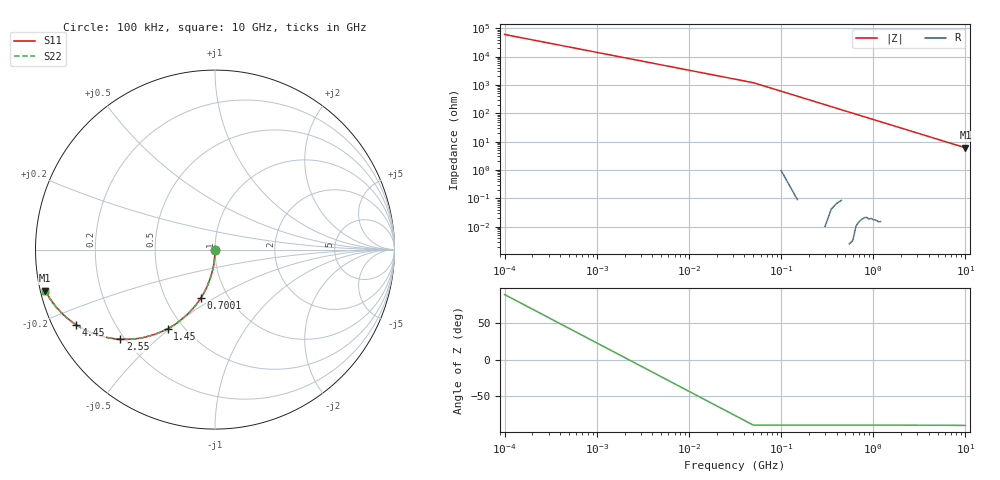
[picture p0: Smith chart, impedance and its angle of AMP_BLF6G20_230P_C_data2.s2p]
! Created Tue Aug  7 13:48:20 2007
# hz S ri R 50
! 2 Port Network Data from SP1.SP block
! freq  reS11  imS11  reS21  imS21  reS12  imS12  reS22  imS22
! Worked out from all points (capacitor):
!   201 points, 100 kHz to 10 GHz, reference 50 ohm
!   read as one part in shunt: C = 2.64 pF near 50.1 MHz
!   lowest |Z| = 6.09 ohm at 10 GHz (marker M1)
!   S11 on the Smith chart (normalised r, x): 100 kHz: 1.00, +0.00; 700.1 MHz: 0.75, -0.43; 1.45 GHz: 0.41, -0.49; 2.55 GHz: 0.18, -0.39; 4.45 GHz: 0.07, -0.25; 10 GHz: 0.01, -0.12
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100000  -2.85e-06 0.000389  1 0.000414  1 0.000414  -2.7e-06 0.000441
5.01e7  -0.000416 -0.0208  0.9996 -0.0209  0.9996 -0.0209  -0.000413 -0.0209
1.001e8  -0.00177 -0.0413  0.9982 -0.0415  0.9982 -0.0415  -0.00178 -0.0415
1.501e8  -0.00386 -0.0618  0.9961 -0.0621  0.9961 -0.0621  -0.00386 -0.0621
2.001e8  -0.00679 -0.082  0.9932 -0.0824  0.9932 -0.0824  -0.00679 -0.0824
2.501e8  -0.0106 -0.1021  0.9894 -0.1026  0.9894 -0.1026  -0.0106 -0.1025
3.001e8  -0.0152 -0.1219  0.9848 -0.1225  0.9848 -0.1225  -0.0152 -0.1224
4.001e8  -0.0267 -0.1606  0.9732 -0.1614  0.9732 -0.1614  -0.0267 -0.1612
5.001e8  -0.0411 -0.1991  0.9588 -0.1986  0.9588 -0.1986  -0.0411 -0.1984
7.001e8  -0.0775 -0.2676  0.9223 -0.2675  0.9223 -0.2675  -0.0775 -0.2672
8.501e8  -0.1103 -0.313  0.8896 -0.3133  0.8896 -0.3133  -0.1103 -0.313
1.0501e9  -0.1588 -0.365  0.841 -0.3657  0.841 -0.3657  -0.1588 -0.3653
1.4501e9  -0.2645 -0.4413  0.7352 -0.4415  0.7352 -0.4415  -0.2644 -0.441
1.7001e9  -0.3309 -0.4702  0.6688 -0.471  0.6688 -0.471  -0.3308 -0.4705
2.0501e9  -0.4183 -0.4937  0.5814 -0.4938  0.5814 -0.4938  -0.4181 -0.4933
2.5501e9  -0.5266 -0.5002  0.473 -0.5  0.473 -0.5  -0.5264 -0.4994
3.3501e9  -0.6575 -0.4752  0.3421 -0.4755  0.3421 -0.4755  -0.6572 -0.4749
4.4501e9  -0.7722 -0.4191  0.2274 -0.4207  0.2274 -0.4207  -0.7719 -0.4201
5.0001e9  -0.8106 -0.3919  0.1889 -0.3932  0.1889 -0.3932  -0.8102 -0.3926
6.7001e9  -0.885 -0.3203  0.1145 -0.3209  0.1145 -0.3209  -0.8846 -0.3203
8.3501e9  -0.923 -0.2679  0.0764 -0.269  0.0764 -0.269  -0.9226 -0.2684
1.00001e10  -0.9452 -0.2292  0.0541 -0.2305  0.0541 -0.2305  -0.9448 -0.2298
